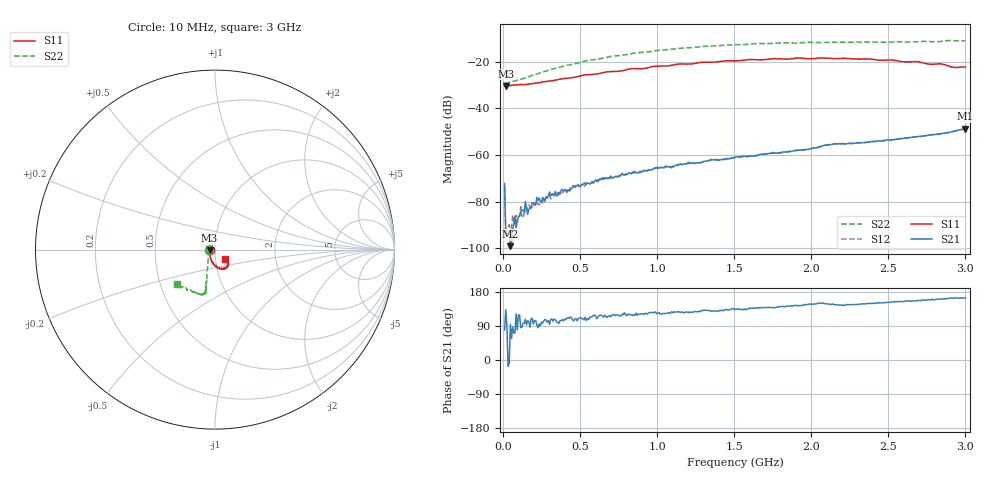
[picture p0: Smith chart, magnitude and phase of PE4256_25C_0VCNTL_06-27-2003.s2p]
!Peregrine Semiconductor Corp.
!S-Parameter Data for Device PE4256 in ISO PATH with TEMP = 25C
!File Created On: 06-27-2003
!Start Frequency = 1.000E+01
!Stop Frequency = 3.000E+03
!Number of Points = 401
# MHZ S DB R 75
!Freq  S11MAG  S11PH  S12MAG  S12PH  S21MAG  S21PH  S22MAG  S22PH
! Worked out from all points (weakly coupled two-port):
!   401 points, 10 MHz to 3 GHz, reference 75 ohm
!   highest |S21| = -48.66 dB at 3 GHz (marker M1); lowest = -99.0 dB at 47.38 MHz (marker M2)
!   lowest |S11| = -30.4 dB at 17.48 MHz (marker M3), VSWR 1.06, Z = 70.6 - j0.259 ohm
!   |S11| at or under -10 dB: start of sweep to end of sweep
!   |S22| runs from -29.1 to -10.9 dB; largest |S21 - S12| = 0.00042
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10  -30.35 -176.0  -72.23 79.2  -73.61 -58.5  -29.08 -175.0
17.48  -30.42 -176.5  -93.58 133.0  -93.50 105.1  -29.11 -173.6
32.43  -30.30 -175.5  -94.30 -16.5  -93.38 52.5  -28.95 -170.1
47.38  -30.17 -173.4  -99.05 94.1  -91.60 78.0  -28.72 -164.5
196.87  -29.33 -150.5  -80.49 94.7  -80.97 106.6  -25.73 -135.2
241.72  -28.90 -145.3  -80.02 89.8  -81.52 103.6  -24.77 -129.8
256.67  -28.67 -143.0  -78.14 97.5  -80.05 100.3  -24.43 -129.1
309  -28.20 -137.6  -77.34 106.8  -78.77 92.6  -23.38 -124.8
361.33  -27.56 -133.5  -76.18 96.6  -76.60 104.0  -22.41 -121.4
391.23  -27.28 -130.5  -75.44 102.9  -75.72 110.2  -21.87 -119.2
421.13  -27.02 -127.6  -74.93 112.4  -75.16 108.8  -21.45 -117.8
451.03  -26.79 -126.2  -74.03 105.7  -73.03 114.4  -21.03 -116.5
510.83  -25.90 -122.4  -72.88 108.8  -72.47 112.6  -20.10 -115.0
660.33  -24.56 -113.1  -69.76 118.1  -69.83 114.5  -18.30 -110.9
1011.65  -21.87 -94.9  -65.70 125.1  -65.42 123.1  -15.08 -105.4
1505  -19.63 -77.4  -60.93 133.1  -61.07 134.0  -12.64 -102.9
2005.82  -18.66 -61.6  -57.10 146.6  -57.12 147.6  -11.67 -104.4
2155.32  -18.63 -57.3  -55.11 145.6  -55.09 146.1  -11.59 -107.1
2506.65  -19.23 -48.1  -53.51 152.1  -53.66 151.6  -11.58 -116.6
2843.02  -20.96 -41.2  -50.85 161.4  -50.88 160.4  -11.28 -130.5
2932.72  -22.48 -42.1  -49.61 163.8  -49.69 164.1  -10.95 -132.4
3000  -22.24 -42.3  -48.66 163.8  -48.68 163.7  -10.97 -137.9
